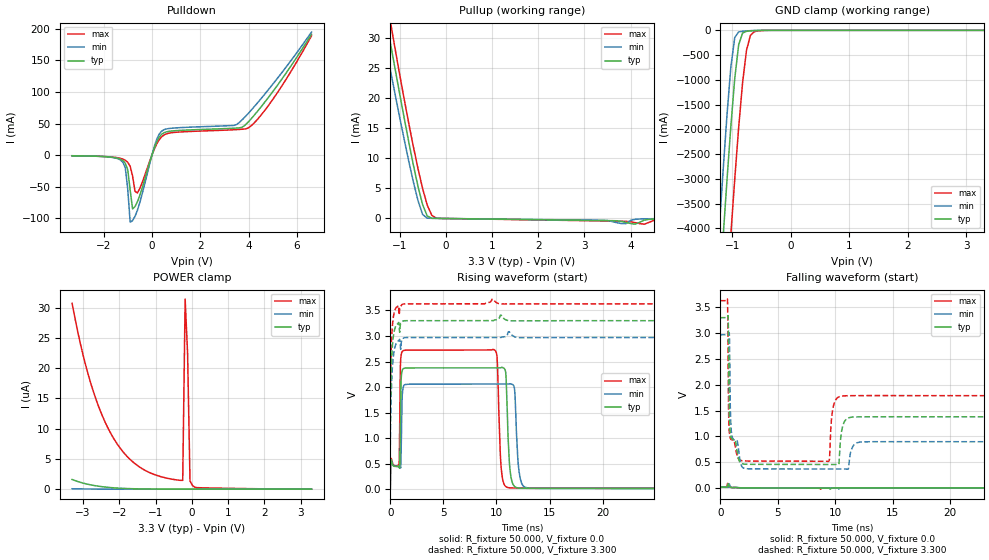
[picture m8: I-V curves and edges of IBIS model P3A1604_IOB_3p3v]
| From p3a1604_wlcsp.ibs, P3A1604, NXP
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[Model] P3A1604_IOB_3p3v
Model_type I/O
Polarity   Non-Inverting
Enable   Active-High
Vinl =  1.394V
Vinh =  1.832V
C_comp   5.400pF   5.000pF   5.900pF
[Model Spec]
Vinh   1.832V   1.554V   2.137V
Vinl   1.394V   1.191V   1.599V
[Temperature Range]   27.000   -40.000   125
[Voltage Range]   3.300V   2.970V   3.630V
[Pullup Reference]   3.300V   2.970V   3.630V
[Pulldown Reference]   0.0V   0.0V   0.0V
[POWER Clamp Reference]   3.300V   2.970V   3.630V
[GND Clamp Reference]   0.0V   0.0V   0.0V
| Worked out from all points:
|   slope of the pulldown table from 0 to 0.495 V, typ, clamps not added: 14 ohm
|   slope of the pullup table from 0 to 0.495 V, typ, clamps not added: 10 kohm
|   GND clamp passes 1 mA (typ) near -0.49 V on its own axis
|   rising waveform, R_fixture 50.000, V_fixture 3.300: 20-80 % time 221ps typ, 242ps min, 202ps max; typ from 1.34 V to 3.3 V
|   falling waveform, R_fixture 50.000, V_fixture 3.300: 20-80 % time 46.5ps typ, 94.2ps min, 36.5ps max; typ from 3.3 V to 1.32 V
[Pulldown]
|Voltage   I(typ)   I(min)   I(max)
-3.3V     -1.04mA    -1.015mA   -1.03mA
-1.2V     -8.769mA   -11.34mA   -6.317mA
-1.1V     -12.97mA   -20.07mA   -8.172mA
-900mV    -55.43mA   -106.3mA   -17.79mA
-800mV    -85.21mA   -103.8mA   -33.05mA
-600mV    -73.9mA    -87.42mA   -60.01mA
100mV     11.47mA    13.69mA    9.571mA
400mV     32.88mA    37.85mA    28.95mA
3.4V      42.65mA    47.08mA    40.18mA
4V        53.11mA    66.71mA    43.38mA
5.1V      105.9mA    117.3mA    93.89mA
6.6V      191.4mA    194.9mA    189.1mA
[Pullup]
|Voltage   I(typ)   I(min)   I(max)
-3.3V     120.2mA    107.2mA    135.2mA
-1.4V     37.63mA    32.64mA    41.82mA
-1.3V     33.39mA    28.65mA    37.25mA
-1.2V     29.17mA    24.69mA    32.75mA
-1.1V     24.98mA    20.77mA    28.33mA
-600mV    5.307mA    2.965mA    8.273mA
-500mV    2.295mA    665.1uA    4.966mA
-400mV    417.2uA    46.79uA    2.206mA
-300mV    42.19uA    26.12uA    510.5uA
-100mV    9.988uA    8.676uA    -96.89nA
4.1V      -937.5uA   -135.3uA   -682.3uA
6.6V      -11.51uA   -6.927uA   -19.35uA
[GND_clamp]
|Voltage   I(typ)   I(min)   I(max)
-3.3V     -45.86A    -44.65A    -48A
-1.223V   -5.431A    -4.072A    -7.72A
-1.156V   -4.222A    -2.873A    -6.498A
-1.089V   -3.052A    -1.738A    -5.299A
-1.022V   -1.947A    -747.6mA   -4.131A
-955mV    -974.3mA   -145.8mA   -3.01A
-888mV    -293.1mA   -31.03mA   -1.966A
-821mV    -55.09mA   -18.69mA   -1.058A
-754mV    -19.87mA   -12.11mA   -403.3mA
-687mV    -11.77mA   -6.785mA   -102mA
-620mV    -6.782mA   -2.859mA   -26.14mA
3.3V      0A         0A         0A
[POWER_clamp]
|Voltage   I(typ)   I(min)   I(max)
-3.3V     1.598uA    68.71nA    30.68uA
-2.931V   899.3nA    33.13nA    20.57uA
-2.529V   452.5nA    13.99nA    13.02uA
-2.06V    184.9nA    4.794nA    7.488uA
-1.524V   57.67nA    1.524nA    4.011uA
-988mV    15.5nA     743.8pA    2.32uA
-251mV    2.823nA    1.719nA    1.46uA
-184mV    2.645nA    757pA      31.4uA
-117mV    7.563nA    458.6pA    22.47uA
-50mV     2.432nA    414pA      1.352uA
17mV      895.5pA    223.2pA    602.8nA
3.3V      0A         0A         0A
[Ramp]
| variable   typ   min   max
dV/dt_r   9.838m/0.378p   7.698m/0.346p   12.959m/0.431p
dV/dt_f   1.189/46.357p   1.284/92.488p   1.137/36.007p
R_load = 50.000
[Rising Waveform]
R_fixture= 50.000
V_fixture= 0.0
V_fixture_min= 0.0
V_fixture_max= 0.0
|time   V(typ)   V(min)   V(max)
0s        1mV        1mV        500uV
820ps     448.4mV    453.4mV    429.8mV
960ps     1.429V     416.8mV    2.465V
1.14ns    2.336V     1.878V     2.699V
9.67ns    2.376V     2.057V     2.738V
10.54ns   2.385V     2.057V     247.2mV
11.72ns   50.25mV    1.911V     23.02mV
12.13ns   21.73mV    341.1mV    22.36mV
13.08ns   17.21mV    18.01mV    21.82mV
1us       16.4mV     12.83mV    21.6mV
[Rising Waveform]
R_fixture= 50.000
V_fixture= 3.300
V_fixture_min= 2.970
V_fixture_max= 3.630
|time   V(typ)   V(min)   V(max)
0s        1.342V     851mV      1.768V
20ps      1.699V     1.268V     2.109V
80ps      2.269V     1.825V     2.685V
260ps     2.942V     2.541V     3.327V
590ps     3.223V     2.869V     3.565V
870ps     3.09V      2.935V     3.496V
980ps     3.245V     2.739V     3.578V
1.3ns     3.298V     2.965V     3.629V
11.17ns   3.3V       3.085V     3.627V
1us       3.3V       2.97V      3.63V
[Falling Waveform]
R_fixture= 50.000
V_fixture= 0.0
V_fixture_min= 0.0
V_fixture_max= 0.0
|time   V(typ)   V(min)   V(max)
0s        16.05mV    11.92mV    21.6mV
540ps     15.75mV    12.89mV    18.81mV
600ps     14.61mV    12.66mV    56.39mV
630ps     28.12mV    11.77mV    85.77mV
680ps     84.77mV    11.18mV    47.88mV
780ps     27.44mV    77.5mV     21.94mV
840ps     17.33mV    32.08mV    13.61mV
1.06ns    4.079mV    6.458mV    8.878mV
9.56ns    -24.39mV   2.517uV    -640nV
1us       18.8nV     3.778nV    3.277uV
[Falling Waveform]
R_fixture= 50.000
V_fixture= 3.300
V_fixture_min= 2.970
V_fixture_max= 3.630
|time   V(typ)   V(min)   V(max)
0s        3.3V       2.969V     3.63V
620ps     3.307V     2.969V     3.631V
710ps     2.801V     2.978V     1.524V
820ps     1.162V     2.32V      997.2mV
1ns       949.6mV    1.013V     932mV
2.48ns    457.2mV    369.8mV    520.6mV
9.44ns    455.4mV    367.2mV    516.4mV
9.97ns    455.3mV    367.2mV    1.676V
11.89ns   1.376V     874mV      1.788V
1us       1.318V     829.6mV    1.736V
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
